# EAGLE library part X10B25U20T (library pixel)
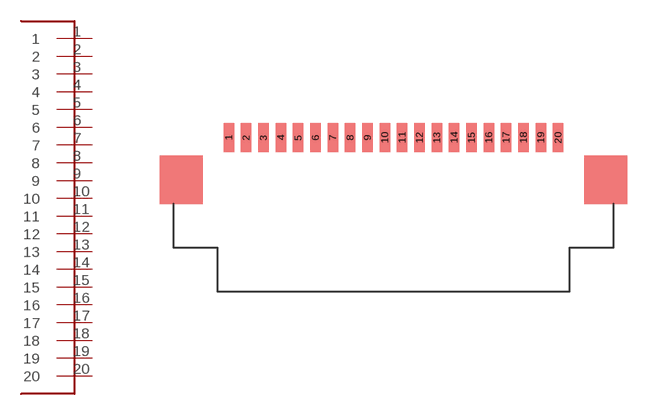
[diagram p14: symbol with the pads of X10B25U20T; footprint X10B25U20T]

Designator prefix -

## X10B25U20T  [X10B25U20T]
1  1
2  2
3  3
4  4
5  5
6  6
7  7
8  8
9  9
10  10
11  11
12  12
13  13
14  14
15  15
16  16
17  17
18  18
19  19
20  20

## Footprint X10B25U20T (pad centres in mm)
smd 0.6 x 1.7: 1 -9.5,-1.016; 2 -8.5,-1.016; 3 -7.5,-1.016; 4 -6.5,-1.016; 5 -5.5,-1.016; 6 -4.5,-1.016; 7 -3.5,-1.016; 8 -2.5,-1.016; 9 -1.5,-1.016; 10 -0.5,-1.016; 11 0.5,-1.016; 12 1.5,-1.016; 13 2.5,-1.016; 14 3.5,-1.016; 15 4.5,-1.016; 16 5.5,-1.016; 17 6.5,-1.016; 18 7.5,-1.016; 19 8.5,-1.016; 20 9.5,-1.016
